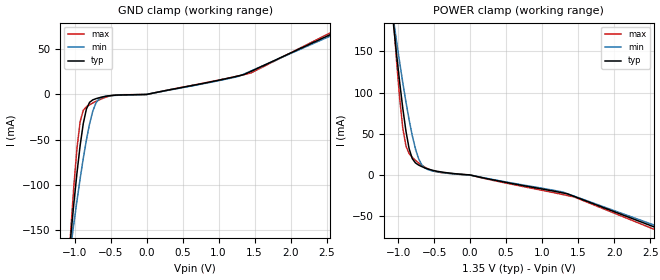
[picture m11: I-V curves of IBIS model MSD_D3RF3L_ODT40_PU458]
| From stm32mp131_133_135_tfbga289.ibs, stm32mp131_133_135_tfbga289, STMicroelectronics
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[Model] MSD_D3RF3L_ODT40_PU458
Model_type   Input
C_comp 2.333pF   2.293pF   2.386pF
Vinh = 810.000mV
Vinl = 540.000mV
[Receiver Thresholds]
Vth   =  0.675V
Vth_min  =  0.6615V
Vth_max  =  0.6885V
Vinh_ac  =  0.160V
Vinh_dc  =  0.090V
Vinl_ac  = -0.160V
Vinl_dc  = -0.090V
Tslew_ac =  5.000ns |Not specified, so set to high value
[Temperature Range]   25.000   125.000   -40.000
[Voltage Range]   1.350V   1.283V   1.450V
[GND Clamp Reference]   0.00V   0.00V   0.00V
[POWER Clamp Reference]   1.350V   1.283V   1.450V
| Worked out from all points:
|   GND clamp passes 1 mA (typ) near -0.47 V on its own axis
|   POWER clamp passes 1 mA (typ) near -0.15 V on its own axis
[GND Clamp]
-1.318V   -415.3mA   -341.2mA   -533.4mA
-1.055V   -159.2mA   -170.4mA   -153.3mA
-1.011V   -121.6mA   -143.6mA   -102.7mA
-966.7mV  -87.17mA   -117.9mA   -59.81mA
-922.7mV  -56.73mA   -93.4mA    -30.19mA
-878.8mV  -32.06mA   -70.69mA   -17.54mA
-834.9mV  -15.93mA   -50.1mA    -13.58mA
-747mV    -5.998mA   -18.51mA   -9.448mA
-615.1mV  -2.826mA   -2.81mA    -4.486mA
200nV     3.415nA    3.262nA    3.445nA
1.45V     25.59mA    25.99mA    23.83mA
2.68V     71mA       69.22mA    73.44mA
[Power Clamp]
-1.33V    441mA      363.7mA    565.9mA
-1.067V   185mA      190.4mA    192.4mA
-1.023V   147.8mA    163.1mA    140.2mA
-978.8mV  112.9mA    136.9mA    93.43mA
-934.9mV  80.8mA     111.8mA    56.63mA
-890.9mV  52.92mA    88.37mA    35.2mA
-847mV    31.8mA     66.82mA    25.89mA
-759.1mV  14.65mA    31.63mA    17.73mA
-671.2mV  10.13mA    12.27mA    11.85mA
-583.3mV  7.191mA    6.461mA    7.386mA
1.438V    -25.81mA   -25.51mA   -26.63mA
2.668V    -66.86mA   -64.43mA   -70mA
